|   Analog Devices INC.
|   IBIS Model of BF527/BF525/BF523
|   Embedded processor
|   289 Pin 12x12 CSP_BGA
[IBIS ver]   3.2
[File name]   bf527_1p8_12x12_evdd.ibs
[File Rev]   1.0
[Date]   02/23/2009
[Source]   From running Hspice on 90nm spice models.
[Notes]
|   Model data reflects 1.8v I/O Operation
|   G16, H17, J22 (actually GND/VDDEXT) are modelled as VDDEXT
|   No models exist for the following pins (Using type NC as
|   a placeholder):
|   XTAL, CLKIN, RTXI, RTXO, USB_ID, USB_DP, USB_XTALOUT,
|   USB_VBUS, USB_DM, VRSEL, USB_XTALIN, VROUT/EXT_WAKE1,
|   SS/PG, USB_RSET, USB_VREF
[Disclaimer]
|   This IBIS model is provided "AS IS, WHERE IS", AND WITH NO WARRANTY OF
|   ANY KIND EITHER EXPRESSED OR IMPLIED, INCLUDING BUT NOT LIMITED TO ANY
|   IMPLIED WARRANTIES OF MERCHANTABILITY AND FITNESS FOR A PARTICULAR
|   PURPOSE.  IN NO EVENT WILL ADI BE LIABLE FOR SPECIAL, COLLATERAL,
|   INCIDENTAL, OR CONSEQUENTIAL DAMAGES IN CONNECTION WITH OR ARISING OUT
|   OF THE USE OF THIS IBIS MODEL, AND IN NO EVENT SHALL ADI'S TOTAL
|   LIABILITY EXCEED $1,000, REGARDLESS OF THE BASIS FOR CLAIM.  ADI
|   RESERVES THE right to make changes to the products and IBIS models
|   without prior notice.
[Copyright]   This model is exclusive property of Analog Devices Inc
|   and is not to be resold or redistributed without the written
|   permission of Analog Devices.
|   Copyright (C)2008 Analog Devices, All Rights Reserved
[Component]   BF527/BF525/BF523
[Manufacturer] ANALOG DEVICES
[Package]
| variable   typ   min   max
R_pkg   167.83m   73m   327m
L_pkg   2.72nH   1.33nH   5.38nH
C_pkg   0.81pF   0.3pF   8.32pF
[Pin]   signal_name   model_name   R_pin   L_pin   C_pin
A1   GND   GND   NA   NA   NA
A2   PG12   prw0408swcdg_25   NA   NA   NA
A3   PG13   prw0408swcdg_25   NA   NA   NA
A4   PG14   prw0812swcdg_25   NA   NA   NA
A5   PG15   prw0408swcdg_3v_25   NA   NA   NA
A6   PPICLK/TMRCLK   prw0408swcdg_25   NA   NA   NA
A7   PF0   prw0408swcdg_25   NA   NA   NA
A8   PF2   prw0812swcdg_25   NA   NA   NA
A9   PF14   prw0408swcdg_25   NA   NA   NA
A10   PF15   prw0408swcdg_25   NA   NA   NA
A11   PH0   prw0408swcdg_25   NA   NA   NA
A12   PH1   prw0408swcdg_25   NA   NA   NA
A13   PH2   prw0408swcdg_25   NA   NA   NA
A14   PH4   prw0408swcdg_25   NA   NA   NA
A15   NC   NC   NA   NA   NA
A16   NC   NC   NA   NA   NA
A17   NC   NC   NA   NA   NA
A18   NC   NC   NA   NA   NA
A19   NC   NC   NA   NA   NA
A20   PF9   prw0812swcdg_25   NA   NA   NA
A21   NC   NC   NA   NA   NA
A22   NC   NC   NA   NA   NA
A23   GND   GND   NA   NA   NA
B1   PG7   prw0408swcdg_25   NA   NA   NA
B2   PG9   prw0812swcdg_25   NA   NA   NA
B3   PG11   prw0408swcdg_25   NA   NA   NA
B4   PG10   prw0812swcdg_25   NA   NA   NA
B5   VDDINT   POWER   NA   NA   NA
B6   GND   GND   NA   NA   NA
B7   PPIFS1/TMR0   prw0408swcdg_25   NA   NA   NA
B8   PF1   prw0408swcdg_25   NA   NA   NA
B9   PF3   prw0408swcdg_25   NA   NA   NA
B10   PF5   prw0812swcdg_25   NA   NA   NA
B11   PF4   prw0408swcdg_25   NA   NA   NA
B12   PF6   prw0408swcdg_25   NA   NA   NA
B13   PF7   prw0408swcdg_25   NA   NA   NA
B14   PH3   prw0408swcdg_25   NA   NA   NA
B15   PF10   prw0408swcdg_25   NA   NA   NA
B16   PF8   prw0408swcdg_25   NA   NA   NA
B17   PF11   prw0408swcdg_25   NA   NA   NA
B18   PF12   prw0408swcdg_25   NA   NA   NA
B19   PF13   prw0812swcdg_25   NA   NA   NA
B20   NC   NC   NA   NA   NA
B21   NC   NC   NA   NA   NA
B22   SCL   piic400kv123   NA   NA   NA
B23   NC   NC   NA   NA   NA
C1   PG8   prw0408swcdg_25   NA   NA   NA
C2   PG6   prw0408swcdg_25   NA   NA   NA
C22   SDA   piic400kv123   NA   NA   NA
C23   NC   NC   NA   NA   NA
D1   PG4   prw0408swcdg_25   NA   NA   NA
D2   PG5   prw0408swcdg_25   NA   NA   NA
D22   NC   NC   NA   NA   NA
D23   NC   NC   NA   NA   NA
E1   BMODE2   prw0408swcdg_25   NA   NA   NA
E2   BMODE3   prw0408swcdg_25   NA   NA   NA
E22   NC   NC   NA   NA   NA
E23   NC   NC   NA   NA   NA
F1   PG3   prw0408swcdg_25   NA   NA   NA
F2   BMODE1   prw0408swcdg_25   NA   NA   NA
F22   NC   NC   NA   NA   NA
F23   NC   NC   NA   NA   NA
G1   PG1   prw0408swcdg_25   NA   NA   NA
G2   BMODE0   prw0408swcdg_25   NA   NA   NA
G7   VDDEXT   POWER   NA   NA   NA
G8   VDDEXT   POWER   NA   NA   NA
G9   VDDEXT   POWER   NA   NA   NA
G10   VDDEXT   POWER   NA   NA   NA
G11   VDDEXT   POWER   NA   NA   NA
G12   VDDEXT   POWER   NA   NA   NA
G13   VDDEXT   POWER   NA   NA   NA
G14   VDDEXT   POWER   NA   NA   NA
G15   VDDEXT   POWER   NA   NA   NA
G16   VDDEXT   POWER   NA   NA   NA
G17   GND   GND   NA   NA   NA
G22   NC   NC   NA   NA   NA
G23   NC   NC   NA   NA   NA
H1   PG2   prw0812swcdg_25   NA   NA   NA
H2   PG0   prw0408swcdg_25   NA   NA   NA
H7   VDDEXT   POWER   NA   NA   NA
H8   VDDINT   POWER   NA   NA   NA
H9   VDDINT   POWER   NA   NA   NA
H10   VDDINT   POWER   NA   NA   NA
H11   VDDINT   POWER   NA   NA   NA
H12   VDDINT   POWER   NA   NA   NA
H13   VDDINT   POWER   NA   NA   NA
H14   VDDINT   POWER   NA   NA   NA
H15   VDDINT   POWER   NA   NA   NA
H16   VDDINT   POWER   NA   NA   NA
H17   VDDEXT   POWER   NA   NA   NA
H22   GND   GND   NA   NA   NA
H23   NC   NC   NA   NA   NA
J1   TDI   prwd0408swcdg_25   NA   NA   NA
J2   EMU   prw0408swcdg_25   NA   NA   NA
J7   VDDMEM   POWER   NA   NA   NA
J8   VDDINT   POWER   NA   NA   NA
J9   GND   GND   NA   NA   NA
J10   GND   GND   NA   NA   NA
J11   GND   GND   NA   NA   NA
J12   GND   GND   NA   NA   NA
J13   GND   GND   NA   NA   NA
J14   GND   GND   NA   NA   NA
J15   GND   GND   NA   NA   NA
J16   VDDINT   POWER   NA   NA   NA
J17   VDDEXT   POWER   NA   NA   NA
J22   VDDEXT   POWER   NA   NA   NA
J23   NC   NC   NA   NA   NA
K1   TDO   prw0408swcdg_25   NA   NA   NA
K2   TRST   prwd0408swcdg_25   NA   NA   NA
K7   VDDMEM   POWER   NA   NA   NA
K8   VDDINT   POWER   NA   NA   NA
K9   GND   GND   NA   NA   NA
K10   GND   GND   NA   NA   NA
K11   GND   GND   NA   NA   NA
K12   GND   GND   NA   NA   NA
K13   GND   GND   NA   NA   NA
K14   GND   GND   NA   NA   NA
K15   GND   GND   NA   NA   NA
K16   VDDINT   POWER   NA   NA   NA
K17   VDDEXT   POWER   NA   NA   NA
K22   PH6   prw0408swcdg_25   NA   NA   NA
K23   PH5   prw0408swcdg_25   NA   NA   NA
L1   TCK   prwd0408swcdg_25   NA   NA   NA
L2   TMS   prwd0408swcdg_25   NA   NA   NA
L7   VDDMEM   POWER   NA   NA   NA
L8   VDDINT   POWER   NA   NA   NA
L9   GND   GND   NA   NA   NA
L10   GND   GND   NA   NA   NA
L11   GND   GND   NA   NA   NA
L12   GND   GND   NA   NA   NA
L13   GND   GND   NA   NA   NA
L14   GND   GND   NA   NA   NA
L15   GND   GND   NA   NA   NA
L16   VDDINT   POWER   NA   NA   NA
L17   VDDEXT   POWER   NA   NA   NA
L22   PH8   prw0408swcdg_25   NA   NA   NA
L23   PH7   prw0408swcdg_25   NA   NA   NA
M1   DATA15   prw1216hcdg_25   NA   NA   NA
M2   DATA14   prw1216hcdg_25   NA   NA   NA
M7   VDDMEM   POWER   NA   NA   NA
M8   VDDINT   POWER   NA   NA   NA
M9   GND   GND   NA   NA   NA
M10   GND   GND   NA   NA   NA
M11   GND   GND   NA   NA   NA
M12   GND   GND   NA   NA   NA
M13   GND   GND   NA   NA   NA
M14   GND   GND   NA   NA   NA
M15   GND   GND   NA   NA   NA
M16   VDDINT   POWER   NA   NA   NA
M17   VDDEXT   POWER   NA   NA   NA
M22   PH10   prw0408swcdg_25   NA   NA   NA
M23   PH12   prw0408swcdg_25   NA   NA   NA
N1   DATA12   prw1216hcdg_25   NA   NA   NA
N2   DATA13   prw1216hcdg_25   NA   NA   NA
N7   VDDMEM   POWER   NA   NA   NA
N8   VDDINT   POWER   NA   NA   NA
N9   GND   GND   NA   NA   NA
N10   GND   GND   NA   NA   NA
N11   GND   GND   NA   NA   NA
N12   GND   GND   NA   NA   NA
N13   GND   GND   NA   NA   NA
N14   GND   GND   NA   NA   NA
N15   GND   GND   NA   NA   NA
N16   VDDINT   POWER   NA   NA   NA
N17   VDDEXT   POWER   NA   NA   NA
N22   PH13   prw0408swcdg_25   NA   NA   NA
N23   PH14   prw0408swcdg_25   NA   NA   NA
P1   DATA9   prw1216hcdg_25   NA   NA   NA
P2   DATA10   prw1216hcdg_25   NA   NA   NA
P7   VDDMEM   POWER   NA   NA   NA
P8   VDDINT   POWER   NA   NA   NA
P9   GND   GND   NA   NA   NA
P10   GND   GND   NA   NA   NA
P11   GND   GND   NA   NA   NA
P12   GND   GND   NA   NA   NA
P13   GND   GND   NA   NA   NA
P14   GND   GND   NA   NA   NA
P15   GND   GND   NA   NA   NA
P16   VDDINT   POWER   NA   NA   NA
P17   VDDEXT   POWER   NA   NA   NA
P22   PH15   prw0408swcdg_25   NA   NA   NA
P23   XTAL   NC   NA   NA   NA
R1   DATA8   prw1216hcdg_25   NA   NA   NA
R2   DATA11   prw1216hcdg_25   NA   NA   NA
R7   VDDMEM   POWER   NA   NA   NA
R8   VDDINT   POWER   NA   NA   NA
R9   GND   GND   NA   NA   NA
R10   GND   GND   NA   NA   NA
R11   GND   GND   NA   NA   NA
R12   GND   GND   NA   NA   NA
R13   GND   GND   NA   NA   NA
R14   GND   GND   NA   NA   NA
R15   GND   GND   NA   NA   NA
R16   VDDINT   POWER   NA   NA   NA
R17   VDDEXT   POWER   NA   NA   NA
R22   PH11   prw0408swcdg_25   NA   NA   NA
R23   CLKIN   NC   NA   NA   NA
T1   DATA7   prw1216hcdg_25   NA   NA   NA
T2   DATA6   prw1216hcdg_25   NA   NA   NA
T7   VDDMEM   POWER   NA   NA   NA
T8   VDDINT   POWER   NA   NA   NA
T9   VDDINT   POWER   NA   NA   NA
T10   VDDINT   POWER   NA   NA   NA
T11   VDDINT   POWER   NA   NA   NA
T12   VDDINT   POWER   NA   NA   NA
T13   VDDINT   POWER   NA   NA   NA
T14   VDDINT   POWER   NA   NA   NA
T15   VDDINT   POWER   NA   NA   NA
T16   VDDINT   POWER   NA   NA   NA
T17   VDDEXT   POWER   NA   NA   NA
T22   GND   GND   NA   NA   NA
T23   PH9   prw0408swcdg_25   NA   NA   NA
U1   DATA5   prw1216hcdg_25   NA   NA   NA
U2   DATA3   prw1216hcdg_25   NA   NA   NA
U7   VDDMEM   POWER   NA   NA   NA
U8   VDDMEM   POWER   NA   NA   NA
U9   VDDMEM   POWER   NA   NA   NA
U10   VDDMEM   POWER   NA   NA   NA
U11   VDDMEM   POWER   NA   NA   NA
U12   VDDMEM   POWER   NA   NA   NA
U13   VDDMEM   POWER   NA   NA   NA
U14   VDDMEM   POWER   NA   NA   NA
U15   VDDMEM   POWER   NA   NA   NA
U16   VDDMEM   POWER   NA   NA   NA
U17   VDDEXT   POWER   NA   NA   NA
U22   NMI   prw0408swcdg_25   NA   NA   NA
U23   RTXI   NC   NA   NA   NA
V1   DATA4   prw1216hcdg_25   NA   NA   NA
V2   DATA1   prw1216hcdg_25   NA   NA   NA
V22   RESET   prw0408swcdg_3v_25   NA   NA   NA
V23   RTXO   NC   NA   NA   NA
W1   DATA2   prw1216hcdg_25   NA   NA   NA
W2   ADDR16   prw1216cdg_25   NA   NA   NA
W22   VDDUSB   POWER   NA   NA   NA
W23   VDDRTC   POWER   NA   NA   NA
Y1   DATA0   prw1216hcdg_25   NA   NA   NA
Y2   ADDR17   prw1216cdg_25   NA   NA   NA
Y22   USB_ID   NC   NA   NA   NA
Y23   VDDUSB   POWER   NA   NA   NA
AA1   ADDR18   prw1216cdg_25   NA   NA   NA
AA2   ADDR15   prw1216cdg_25   NA   NA   NA
AA22   USB_DP   NC   NA   NA   NA
AA23   USB_XTALOUT NC   NA   NA   NA
AB1   ADDR19   prw1216cdg_25   NA   NA   NA
AB2   ADDR13   prw1216cdg_25   NA   NA   NA
AB3   ADDR11   prw1216cdg_25   NA   NA   NA
AB4   ADDR7   prw1216cdg_25   NA   NA   NA
AB5   ADDR8   prw1216cdg_25   NA   NA   NA
AB6   ADDR6   prw1216cdg_25   NA   NA   NA
AB7   ADDR3   prw1216cdg_25   NA   NA   NA
AB8   ADDR1   prw1216cdg_25   NA   NA   NA
AB9   ABE0/SDQM0  prw1216cdg_25   NA   NA   NA
AB10   SWE   prw1216cdg_25   NA   NA   NA
AB11   VPPOTP   POWER   NA   NA   NA
AB12   SRAS   prw1216cdg_25   NA   NA   NA
AB13   SCKE   prw1216cdg_25   NA   NA   NA
AB14   AWE   prw1216cdg_25   NA   NA   NA
AB15   AMS3   prw1216cdg_25   NA   NA   NA
AB16   AMS1   prw1216cdg_25   NA   NA   NA
AB17   ARE   prw1216cdg_25   NA   NA   NA
AB18   CLKOUT   prw1624cdg_25   NA   NA   NA
AB19   CLKBUF   prw0408swcdg_3v_25   NA   NA   NA
AB20   USB_VBUS   NC   NA   NA   NA
AB21   USB_DM   NC   NA   NA   NA
AB22   VRSEL   NC   NA   NA   NA
AB23   USB_XTALIN  NC   NA   NA   NA
AC1   GND   GND   NA   NA   NA
AC2   ADDR14   prw1216cdg_25   NA   NA   NA
AC3   ADDR12   prw1216cdg_25   NA   NA   NA
AC4   ADDR10   prw1216cdg_25   NA   NA   NA
AC5   ADDR9   prw1216cdg_25   NA   NA   NA
AC6   ADDR5   prw1216cdg_25   NA   NA   NA
AC7   ADDR4   prw1216cdg_25   NA   NA   NA
AC8   ADDR2   prw1216cdg_25   NA   NA   NA
AC9   ABE1/SDQM1  prw1216cdg_25   NA   NA   NA
AC10   SA10   prw1216cdg_25   NA   NA   NA
AC11   SCAS   prw1216cdg_25   NA   NA   NA
AC12   VDDOTP   POWER   NA   NA   NA
AC13   SMS   prw1216cdg_25   NA   NA   NA
AC14   ARDY   prw1216cdg_25   NA   NA   NA
AC15   AOE   prw1216cdg_25   NA   NA   NA
AC16   AMS2   prw1216cdg_25   NA   NA   NA
AC17   AMS0   prw1216cdg_25   NA   NA   NA
AC18  VROUT/EXT_WAKE1 NC   NA   NA   NA
AC19   EXT_WAKE2   prw0408swcdg_3v_25   NA   NA   NA
AC20   SS/PG   NC   NA   NA   NA
AC21   USB_RSET   NC   NA   NA   NA
AC22   USB_VREF   NC   NA   NA   NA
AC23   GND   GND   NA   NA   NA
[Model Selector]   prw0408swcdg_25
COUT_8 8mA buffer
[Model Selector]   prwd0408swcdg_25
EOUT_8 8mA buffer
[Model Selector]   prw0408swcdg_3v_25
FOUT_8 8mA buffer
[Model Selector]   prw0812swcdg_25
IOUT_12 12mA buffer
[Model Selector]   prw1216cdg_25
MOUT_16 16mA buffer
[Model Selector]   prw1216hcdg_25
NOUT_16 16mA buffer
[Model Selector]   prw1624cdg_25
QOUT_24 24mA buffer
[Model Selector]   piic400kv123
twi_s5 Vbus 1.8V
twi_s6 Vbus 2.5V
twi_s7 Vbus 3.3V
| Models and submodels in the file (10): twi_s5 (I/O_open_drain), twi_s6 (I/O_open_drain), twi_s7 (I/O_open_drain), COUT_8 (I/O), FOUT_8 (I/O), IOUT_12 (I/O), MOUT_16 (I/O), NOUT_16 (I/O), EOUT_8 (I/O), QOUT_24 (I/O)
